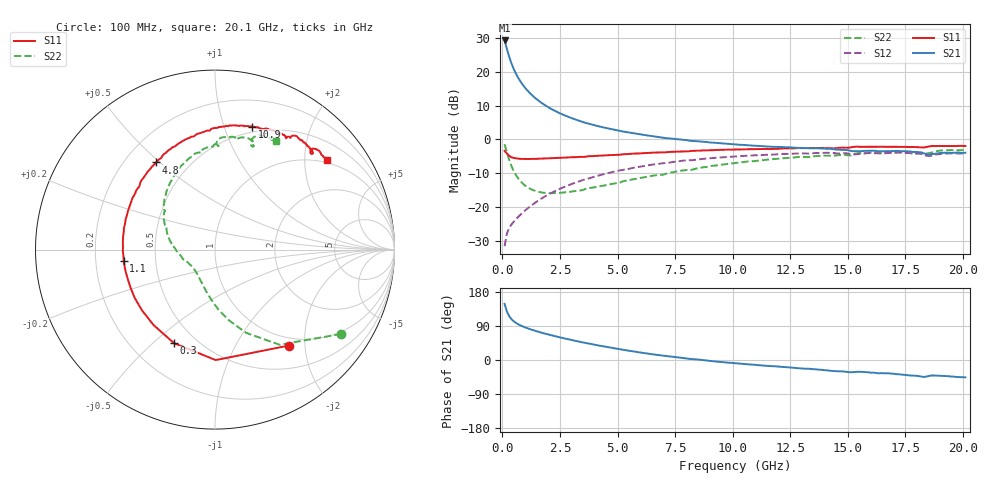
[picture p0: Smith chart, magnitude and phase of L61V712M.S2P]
!  Infineon Technologies AG
! BFR380L3 , PF131585-7, No.6, Th 09.10.01, soldered on pcb-board, measured with PP GSG850
!  Vce=1.75 V,  Ic=12.5 mA
! Common Emitter S-Parameters:  15. November 2001
#  GHz  S  MA  R  50
! f  S11  S21  S12  S22
! GHz  Mag  Ang  Mag  Ang  Mag  Ang  Mag  Ang
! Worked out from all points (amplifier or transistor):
!   201 points, 100 MHz to 20.1 GHz, reference 50 ohm
!   highest |S21| = 29.3 dB at 100 MHz (marker M1)
!   |S21| within 3 dB of that: start of sweep to 220.6 MHz
!   unconditionally stable (mu >= 1): 1.661 GHz to 4.606 GHz
!   at 3.4 GHz: K = 1.03, MAG = 7.8 dB, |S12| = -12.3 dB
!   at 10.1 GHz: K = 0.96, MSG = 1.8 dB, |S12| = -5.1 dB
!   at 20.1 GHz: K = 0.99, MSG = 0.1 dB, |S12| = -4.2 dB
!   S11 on the Smith chart (normalised r, x): 100 MHz: 0.86, -1.69; 300 MHz: 0.38, -0.58; 1.1 GHz: 0.32, -0.06; 4.8 GHz: 0.33, +0.49; 10.9 GHz: 0.44, +1.25; 20.1 GHz: 0.93, +2.54
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0.1  0.6749 -52.4  29.21 148.2  0.02609 65.5  0.8463 -33.7
0.2  0.6155 -89.7  21.86 127.6  0.04021 54.9  0.641 -55.8
0.3  0.569 -113.7  16.69 115.5  0.04883 50.8  0.4946 -69.6
0.4  0.542 -129.3  13.28 107.6  0.05479 49.8  0.3995 -79.1
0.5  0.529 -140.4  10.94 101.9  0.06032 50.4  0.3363 -86.5
0.6  0.5221 -148.8  9.278 97.7  0.06576 51.5  0.2926 -92.3
0.7  0.5164 -155.3  8.054 94.0  0.07119 52.6  0.2606 -97.5
0.8  0.513 -160.7  7.103 90.9  0.07712 54.1  0.2369 -102.0
0.9  0.5127 -165.5  6.353 88.3  0.08296 55.0  0.2187 -106.1
1.1  0.5126 -172.9  5.259 83.6  0.09498 56.7  0.1946 -113.5
1.3  0.5137 -179.0  4.483 79.4  0.1072 57.8  0.1788 -119.6
1.5  0.5146 175.7  3.914 75.6  0.1199 58.5  0.1693 -125.2
2  0.5212 164.9  2.984 67.3  0.1522 58.6  0.1598 -137.0
2.6  0.5323 154.2  2.346 58.3  0.1912 57.1  0.1623 -148.6
3.5  0.549 140.4  1.804 46.3  0.2496 52.9  0.1771 -161.8
4.8  0.586 124.0  1.402 31.4  0.3282 45.4  0.2195 179.6
6.8  0.6383 102.9  1.08 12.9  0.4355 32.1  0.2969 155.5
10.1  0.7066 77.9  0.8405 -8.6  0.5571 10.7  0.4459 124.5
10.9  0.716 73.1  0.8066 -12.4  0.5773 5.8  0.4741 117.3
13.5  0.7423 60.4  0.7377 -24.2  0.6222 -9.8  0.5573 97.5
16.8  0.7746 48.0  0.6704 -35.4  0.6269 -25.6  0.6419 76.7
20.1  0.7975 38.8  0.6325 -45.9  0.6199 -39.1  0.6941 60.7
